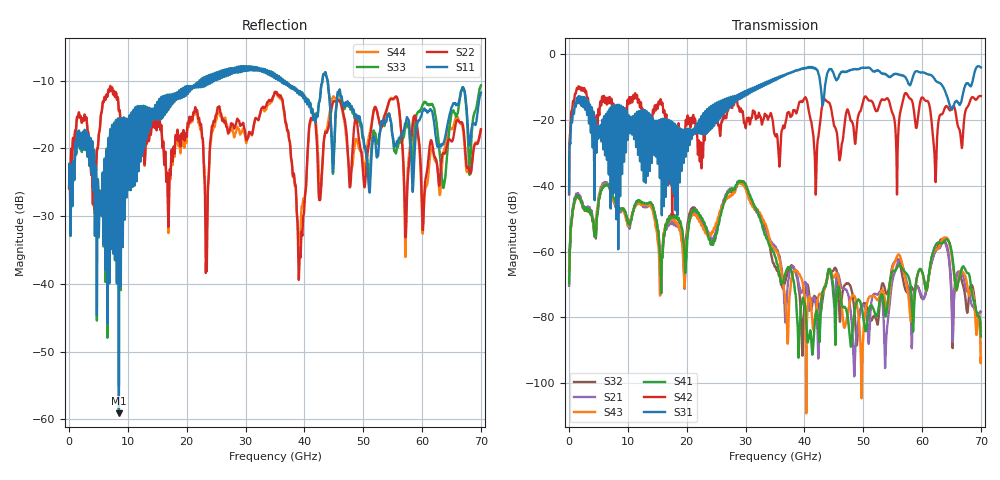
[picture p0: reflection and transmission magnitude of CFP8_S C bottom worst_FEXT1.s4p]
! AWR Design Environment (8415) Tue Jan 08 14:13:14 2019
! Document = 'CFP8 Channel_S_2'
! nPorts: 4, nXvals: 7001
# HZ S DB R 50
!Freq DBS11 AngS11 DBS12 AngS12 DBS13 AngS13 DBS14 AngS14
!	DBS21 AngS21 DBS22 AngS22 DBS23 AngS23 DBS24 AngS24
!	DBS31 AngS31 DBS32 AngS32 DBS33 AngS33 DBS34 AngS34
!	DBS41 AngS41 DBS42 AngS42 DBS43 AngS43 DBS44 AngS44
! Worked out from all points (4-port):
!   7000 points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, 10 MHz to 70 GHz, reference 50 ohm
!   strongest paths, dB at 10 MHz, 17.51 GHz, 35.01 GHz, 52.51 GHz, 70 GHz:
!     S31: -42.3, -25.6, -7.5, -4.9, -4.0
!     S42: -42.6, -46.4, -24.6, -16.7, -12.8
!     S41: -69.7, -49.7, -61.6, -78.3, -85.7
!     S43: -65.9, -50.4, -59.4, -74.7, -92.3
!     S21: -70.4, -51.6, -58.6, -73.0, -78.2
!     S32: -66.0, -49.0, -64.7, -81.7, -84.0
!   lowest |S11| = -59.1 dB at 8.47 GHz (marker M1), VSWR 1.00, Z = 50 + j0.109 ohm
!   |S11| at or under -10 dB: start of sweep to 22.19 GHz; 36.39 GHz to 43.06 GHz (6.667 GHz wide, 16.8 % of centre); 43.96 GHz to end of sweep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
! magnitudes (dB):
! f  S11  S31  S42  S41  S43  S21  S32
! 10 MHz  -25.6  -42.3  -42.6  -69.7  -65.9  -70.4  -66.0
! 1.6 GHz  -18.4  -12.8  -9.8  -43.2  -43.4  -42.4  -42.9
! 8.47 GHz  -59.1  -16.4  -19.9  -46.9  -47.0  -48.1  -47.6
! 29.58 GHz  -7.9  -11.9  -18.4  -38.8  -39.8  -38.8  -39.0
! 40.62 GHz  -12.9  -4.2  -16.0  -87.3  -75.1  -74.9  -70.4
! 64.03 GHz  -17.9  -11.7  -15.9  -56.3  -55.7  -57.9  -57.3
! 70 GHz  -11.8  -4.0  -12.8  -85.7  -92.3  -78.2  -84.0
